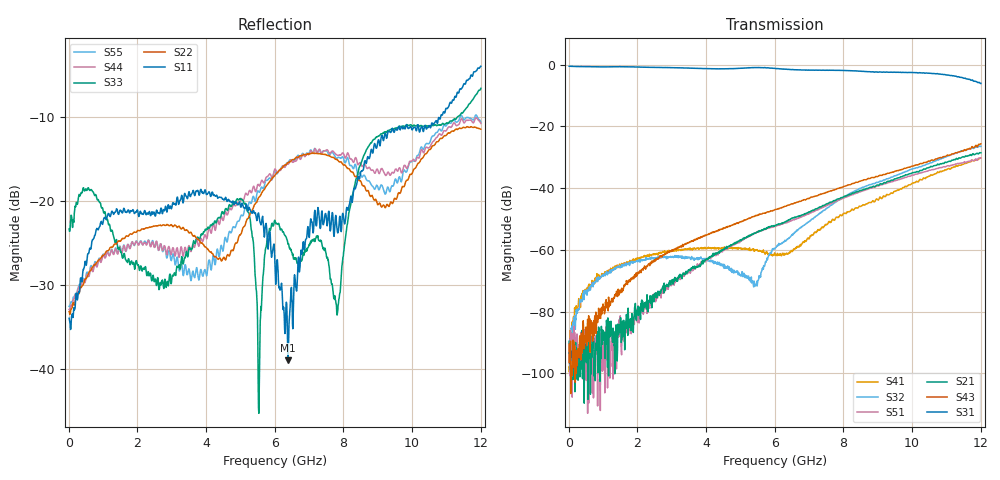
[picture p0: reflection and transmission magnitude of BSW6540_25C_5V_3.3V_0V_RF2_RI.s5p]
! Agilent Technologies	N5230C	MY49001333	A.09.33.09
!	Test time	=	2026-05-06 10:00
!	Product	=	BSW6540
!	Temp	=	25C
!	VDD	=	5
!	Control_High	=	3.3
!	Control_Low	=	0
!	Logic	=	RF2
!	Port1	=	RFC
!	Port2	=	RF1
!	Port3	=	RF2
!	Port4	=	RF3
!	Port5	=	RF4
!	V1	=	3.3 / 0
!	V2	=	3.3 / 0
!S5P File: Measurements: <S11,S12,S13,S14,S15>,
!<S21,S22,S23,S24,S25>,
!<S31,S32,S33,S34,S35>,
!<S41,S42,S43,S44,S45>,
!<S51,S52,S53,S54,S55>;
# HZ S RI R 50
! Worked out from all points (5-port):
!   1201 points, 10 MHz to 12.01 GHz, reference 50 ohm
!   strongest paths, dB at 10 MHz, 3.01 GHz, 6.01 GHz, 9.01 GHz, 12.01 GHz:
!     S31: -0.5, -1.0, -1.2, -2.4, -6.1
!     S43: -96.5, -60.2, -47.0, -36.2, -25.7
!     S21: -89.6, -69.8, -52.1, -39.0, -28.6
!     S51: -94.7, -71.0, -52.4, -39.3, -30.3
!     S32: -93.7, -62.2, -59.4, -38.1, -26.4
!     S41: -97.9, -60.1, -61.4, -43.8, -30.3
!   lowest |S11| = -39.0 dB at 6.39 GHz (marker M1), VSWR 1.02, Z = 49.4 + j0.948 ohm
!   |S11| at or under -10 dB: start of sweep to 10.84 GHz
